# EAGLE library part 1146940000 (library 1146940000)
PCB plug-in connector, male header, open side, THT solder connection, 5.08 mm, Number of poles: 12, 90, Solder pin length: 3.2 mm, tinned, orange, Box Source: Datasheet
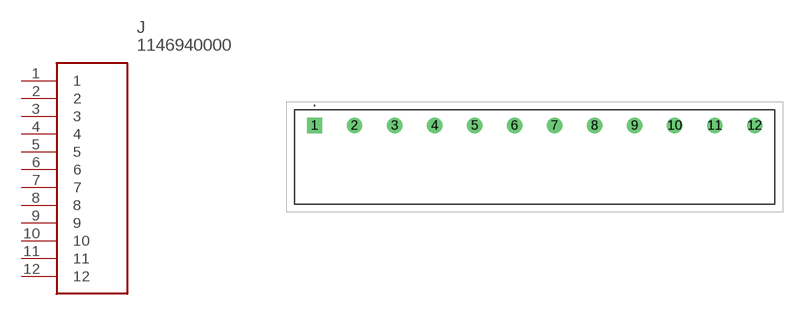
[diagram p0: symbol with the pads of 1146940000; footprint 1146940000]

Designator prefix J

## 1146940000 (Description: PCB plug-in connector, male header, open side, THT solder connection, 5.08 mm, Number of poles: 12, 90, Solder pin length: 3.2 mm, tinned, orange, Box; Height: 8.4mm; Manufacturer_Name: Weidmuller; Manufacturer_Part_Number: 1146940000)  [1146940000]
1  1
2  2
3  3
4  4
5  5
6  6
7  7
8  8
9  9
10  10
11  11
12  12

## Footprint 1146940000 (pad centres in mm)
1146940000-1
drill 1.3 pad 1.95 square: 1 0,0
drill 1.3 pad 1.95: 2 5.08,0; 3 10.16,0; 4 15.24,0; 5 20.32,0; 6 25.4,0; 7 30.48,0; 8 35.56,0; 9 40.64,0; 10 45.72,0; 11 50.8,0; 12 55.88,0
